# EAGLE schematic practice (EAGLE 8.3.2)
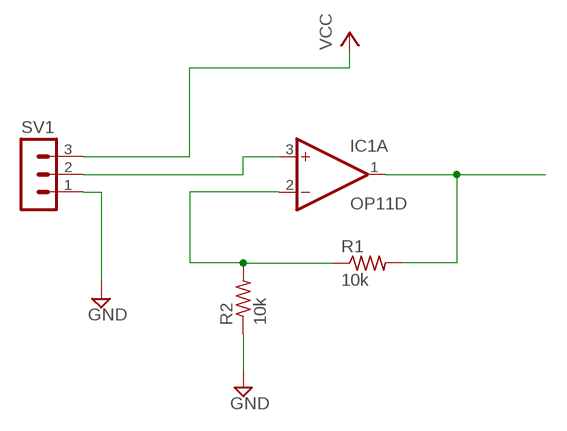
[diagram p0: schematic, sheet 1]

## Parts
IC1  OP11D  [SO14]
R1  10k  R-US_R0805  [R0805]
R2  10k  R-US_R0805  [R0805]
SV1  MA03-1  [MA03-1]

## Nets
GND: R2.1 SV1.1
N$1: IC1.1(A:OUT) R1.2
N$2: IC1.2(A:-IN) R1.1 R2.2
N$5: IC1.3(A:+IN) SV1.2
VCC: SV1.3
Unconnected: IC1.5(B:+IN) IC1.6(B:-IN) IC1.7(B:OUT) IC1.8(C:OUT) IC1.9(C:-IN) IC1.10(C:+IN) IC1.12(D:+IN) IC1.13(D:-IN) IC1.14(D:OUT)

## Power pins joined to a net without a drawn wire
V+: IC1.4(P:V+)
V-: IC1.11(P:V-)

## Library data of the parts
IC1 = linear:OP11: Quad Low-Offset Low-Power OP AMP The OP-11 is pin compatible with the OP-400 , LM148, HA4741, RM4156, and LT1014 operational amplifiers source http://products.analog.com/products/info.asp?product=OP400
R1 R2 = rcl:R-US_: RESISTOR, American symbol
SV1 = con-lstb:MA03-1: PIN HEADER; OC_FARNELL: unknown; OC_NEWARK: unknown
